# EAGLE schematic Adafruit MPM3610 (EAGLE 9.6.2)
COMPANY: ADAFRUIT INDUSTRIES; DRAWN: KTOWN; REV: A
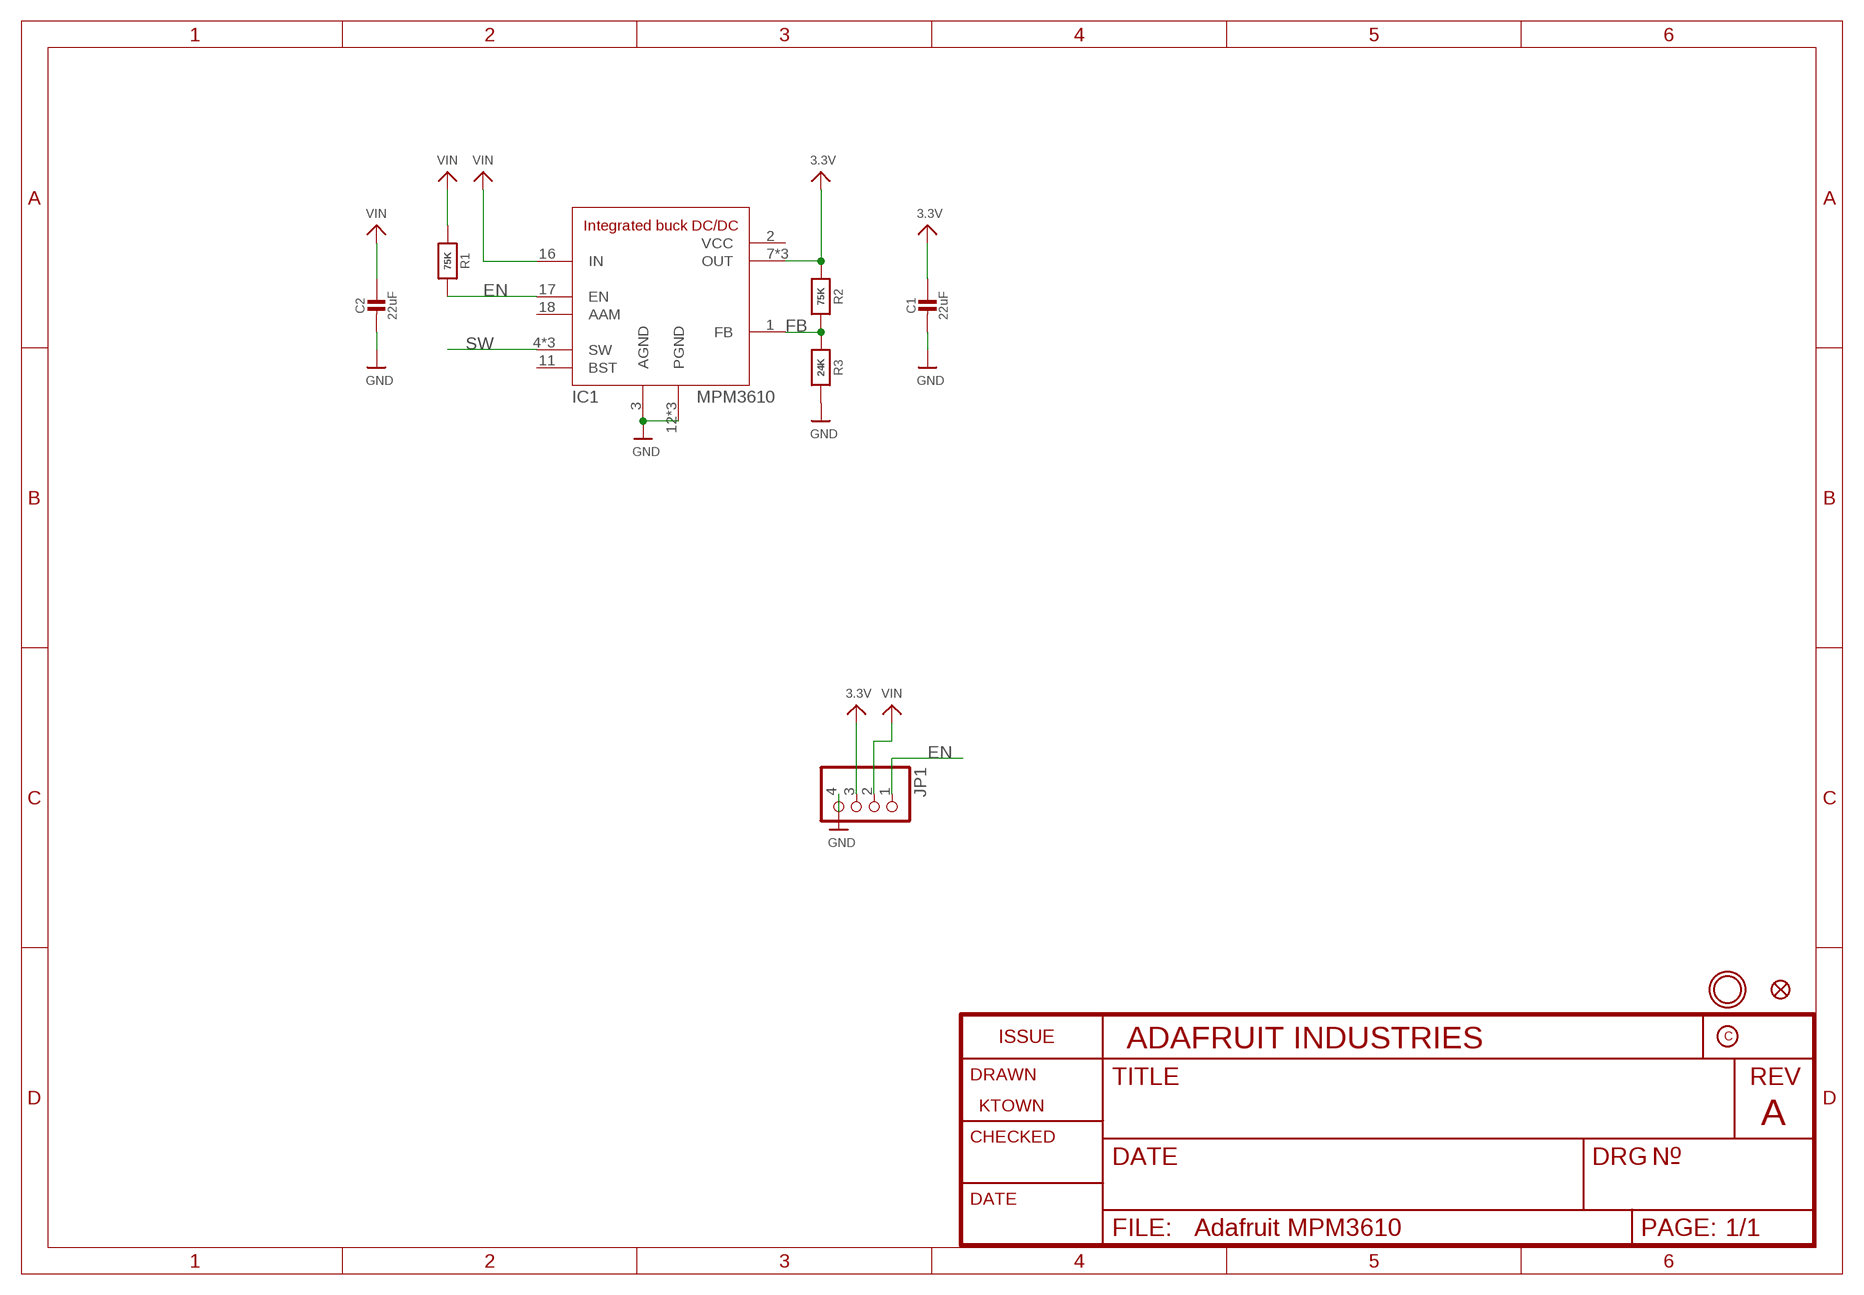
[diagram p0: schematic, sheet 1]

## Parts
C1  22uF  CAP_CERAMIC0805-NOOUTLINE  [0805-NO]
C2  22uF  CAP_CERAMIC0805-NOOUTLINE  [0805-NO]
FID1  FIDUCIAL_1MM  [FIDUCIAL_1MM]
IC1  MPM3610  [MPM3610]
JP1  HEADER-1X4ROUND  [1X04_ROUND]
R1  75K  RESISTOR_0603_NOOUT  [0603-NO]
R2  75K  RESISTOR_0603_NOOUT  [0603-NO]
R3  24K  RESISTOR_0603_NOOUT  [0603-NO]
U$9  MOUNTINGHOLE2.5  [MOUNTINGHOLE_2.5_PLATED]

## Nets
3.3V: C1.1 IC1.7(OUT) IC1.8(OUT) IC1.9(OUT) JP1.3 R2.1
EN: IC1.17(EN) JP1.1 R1.2
FB: IC1.1(FB) R2.2 R3.1
GND: C1.2 C2.2 IC1.3(AGND) IC1.12(PGND) IC1.13(PGND) IC1.14(PGND) JP1.4 R3.2
SW: IC1.4(SW) IC1.5(SW) IC1.6(SW)
VIN: C2.1 IC1.16(IN) JP1.2 R1.1
Unconnected: IC1.11(BST) IC1.18(AAM)

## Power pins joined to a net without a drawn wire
VCC: IC1.2(VCC)

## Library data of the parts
C1 C2 = microbuilder:CAP_CERAMIC: Ceramic Capacitors
FID1 = microbuilder:FIDUCIAL: Fiducial Alignment Points; BOM: EXCLUDE
IC1 = microbuilder:MPM3610
JP1 = microbuilder:HEADER-1X4: PIN HEADER
R1-R3 = microbuilder:RESISTOR: Resistors
U$9 = microbuilder:MOUNTINGHOLE: Mounting Hole; BOM: EXCLUDE

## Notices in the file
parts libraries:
microbuilder: This work is placed in the public domain, and may be freely used for commercial and non-commercial work with the following conditions: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
